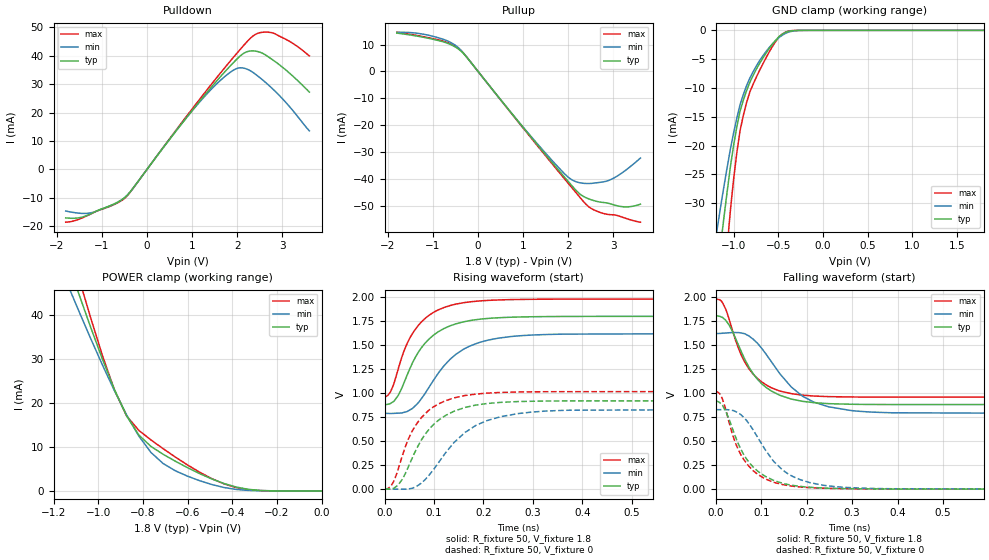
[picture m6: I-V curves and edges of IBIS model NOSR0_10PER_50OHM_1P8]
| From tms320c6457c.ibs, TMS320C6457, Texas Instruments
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|   Model Cell NOSR0_10PER_50OHM_1P8
|NOSR0_10PER_50OHM_1P8
[Model]   NOSR0_10PER_50OHM_1P8
Model_type   3-state
Polarity   Non-Inverting
Enable   Active-Low
Cref =  15.0000pF
Rref =  100.0000M
Vref =  0V
Vmeas =  0.9
C_comp   1.89p   1.72p   2.18p
[Model Spec]
Rref 50 NA NA
Vref 0.9 0.81 0.99
[Temperature Range]   25   125   -40
[Voltage Range]   1.8   1.62   1.98
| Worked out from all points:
|   slope of the pulldown table from 0 to 0.27 V, typ, clamps not added: 47.1 ohm
|   slope of the pullup table from 0 to 0.27 V, typ, clamps not added: 47.4 ohm
|   GND clamp passes 1 mA (typ) near -0.48 V on its own axis
|   POWER clamp passes 1 mA (typ) near -0.39 V on its own axis
|   rising waveform, R_fixture 50, V_fixture 1.8: 20-80 % time 66.5ps typ, 82.3ps min, 59ps max; typ from 0.882 V to 1.8 V
|   rising waveform, R_fixture 50, V_fixture 0: 20-80 % time 70.4ps typ, 91.1ps min, 60.7ps max; typ from 0.001 V to 0.92 V
|   falling waveform, R_fixture 50, V_fixture 1.8: 20-80 % time 70.1ps typ, 92.5ps min, 60.6ps max; typ from 1.8 V to 0.882 V
|   falling waveform, R_fixture 50, V_fixture 0: 20-80 % time 64.5ps typ, 81.1ps min, 57.1ps max; typ from 0.92 V to 0.001 V
| Nom Voltages:
|   BIAS2=0.9, BIASFET=0, VDD=1.1, VDDS=1.8, BUS_BIAS1=0, BUS_BIAS3=0,
|   VSS=0, VSSS=0
| Min Voltages:
|   BIAS2=0.81, BIASFET=0, VDD=0.99, VDDS=1.62, BUS_BIAS1=0, BUS_BIAS3=0,
|   VSS=0, VSSS=0
| Max Voltages:
|   BIAS2=0.99, BIASFET=0, VDD=1.21, VDDS=1.98, BUS_BIAS1=0, BUS_BIAS3=0,
|   VSS=0, VSSS=0
[POWER_clamp]
|   voltage   I(typ)   I(min)   I(max)
-1.8V     156mA      133.5mA    181.7mA
-1.127V   50.87mA    45.88mA    55.74mA
-1.109V   48.19mA    43.68mA    52.51mA
-1.073V   42.88mA    39.33mA    46.15mA
-1.055V   40.27mA    37.18mA    43.01mA
-927.3mV  23.11mA    22.83mA    22.99mA
-872.7mV  17.08mA    17.31mA    17.08mA
-818.2mV  12.73mA    12.5mA     13.8mA
-763.6mV  10.13mA    8.758mA    11.61mA
-600mV    5.297mA    3.359mA    5.911mA
-381.8mV  881.1uA    334.9uA    769uA
0V        130.3nA    147.3nA    381.2nA
[Pulldown]
|   voltage   I(typ)   I(min)   I(max)
-1.8V     -17.05mA   -14.61mA   -18.56mA
-1.527V   -17.06mA   -15.36mA   -17.63mA
-1.255V   -15.7mA    -15.3mA    -15.76mA
-490.9mV  -9.876mA   -9.852mA   -10.12mA
1.2V      24.63mA    24.33mA    25.37mA
1.691V    33.76mA    32.26mA    35.17mA
2.018V    39.25mA    35.69mA    41.38mA
2.291V    41.73mA    34.78mA    46.18mA
2.455V    41.53mA    32.94mA    47.93mA
2.673V    39.85mA    30.05mA    48.36mA
3.164V    33.87mA    22.08mA    45.09mA
3.6V      27.27mA    13.61mA    39.99mA
[Pullup]
|   voltage   I(typ)   I(min)   I(max)
-1.8V     14.26mA    14.49mA    14.63mA
-1.364V   13.18mA    14.23mA    13.4mA
-927.3mV  11.68mA    12.75mA    11.91mA
-600mV    9.93mA     10.72mA    10.21mA
-381.8mV  7.614mA    7.959mA    7.791mA
1.309V    -27.19mA   -26.85mA   -27.53mA
1.909V    -39.21mA   -37.96mA   -39.84mA
2.127V    -43.46mA   -40.78mA   -44.26mA
2.455V    -47.47mA   -41.74mA   -50.41mA
2.891V    -49.11mA   -40.62mA   -53.29mA
3.273V    -50.45mA   -36.79mA   -54.71mA
3.6V      -49.43mA   -32.25mA   -56.14mA
[GND_clamp]
|   voltage   I(typ)   I(min)   I(max)
-1.8V     -137.1mA   -107.1mA   -189.7mA
-1.182V   -42.18mA   -34.28mA   -58.62mA
-1.109V   -32.61mA   -27.18mA   -44.51mA
-1.073V   -28.08mA   -23.86mA   -37.8mA
-1.036V   -23.72mA   -20.65mA   -31.33mA
-963.6mV  -16.74mA   -15.21mA   -21.21mA
-927.3mV  -13.99mA   -12.88mA   -17.38mA
-854.5mV  -10.47mA   -9.599mA   -12.54mA
-781.8mV  -7.837mA   -7.198mA   -9.373mA
-600mV    -3.116mA   -2.961mA   -3.703mA
-418.2mV  -354.7uA   -522.3uA   -297.6uA
1.8V      130.3nA    2.912uA    201.9nA
[Ramp]
| variable   typ   min   max
dV/dt_f 0.46193803/54.999737p  0.4204107/72.789897p 0.51208619/47.43615p
dV/dt_r 0.46230814/55.152557p 0.41704691/71.272487p 0.51005622/47.439453p
R_load = 50
[Rising Waveform]
R_fixture = 50
V_fixture = 1.8
V_fixture_min = 1.62
V_fixture_max = 1.98
|   time   V(typ)   V(min)   V(max)
0s        881.8mV    790.3mV    958.1mV
12.09ps   894.1mV    787.9mV    1.016V
27.69ps   977.9mV    791.7mV    1.255V
45.68ps   1.189V     808.7mV    1.519V
67.59ps   1.421V     896.7mV    1.702V
108ps     1.637V     1.203V     1.866V
160.1ps   1.743V     1.459V     1.942V
229.8ps   1.785V     1.572V     1.97V
329.6ps   1.797V     1.611V     1.979V
1.185ns   1.8V       1.62V      1.98V
[Rising Waveform]
R_fixture = 50
V_fixture = 0
V_fixture_min = 0
V_fixture_max = 0
|   time   V(typ)   V(min)   V(max)
0s        668uV      196.3uV    466.7uV
12.46ps   2.727mV    0V         30.23mV
27.69ps   44.51mV    0V         212.9mV
48.99ps   243.9mV    3.035mV    531.9mV
73.79ps   507.6mV    60.68mV    740.7mV
109.1ps   718.3mV    276.4mV    887.8mV
162.9ps   851.1mV    591mV      975.6mV
235.2ps   904.2mV    755.2mV    1.007V
329.6ps   917.8mV    814.4mV    1.015V
1.185ns   920.1mV    827.8mV    1.017V
[Falling Waveform]
R_fixture = 50
V_fixture = 1.8
V_fixture_min = 1.62
V_fixture_max = 1.98
|   time   V(typ)   V(min)   V(max)
0s        1.799V     1.62V      1.98V
14.89ps   1.789V     1.624V     1.943V
29.09ps   1.712V     1.629V     1.776V
57.09ps   1.423V     1.625V     1.386V
82.69ps   1.2V       1.561V     1.196V
122.7ps   1.022V     1.325V     1.055V
166.1ps   938.7mV    1.065V     995.4mV
215.8ps   901.1mV    907mV      970.2mV
333.9ps   882.7mV    805.4mV    959.5mV
1.185ns   881.7mV    790.9mV    958.5mV
[Falling Waveform]
R_fixture = 50
V_fixture = 0
V_fixture_min = 0
V_fixture_max = 0
|   time   V(typ)   V(min)   V(max)
0s        920.5mV    828.2mV    1.017V
9.494ps   898.2mV    828.2mV    988mV
21.89ps   813.9mV    828.2mV    832.2mV
38.69ps   606.3mV    819.2mV    543.9mV
60.99ps   365.1mV    751.1mV    314.1mV
92.69ps   186.6mV    536.5mV    153.2mV
147.2ps   61.56mV    199.9mV    48.35mV
206.7ps   20.58mV    69.19mV    16.5mV
321ps     4.199mV    11.35mV    4.177mV
1.185ns   998.2uV    1.056mV    632.9uV
